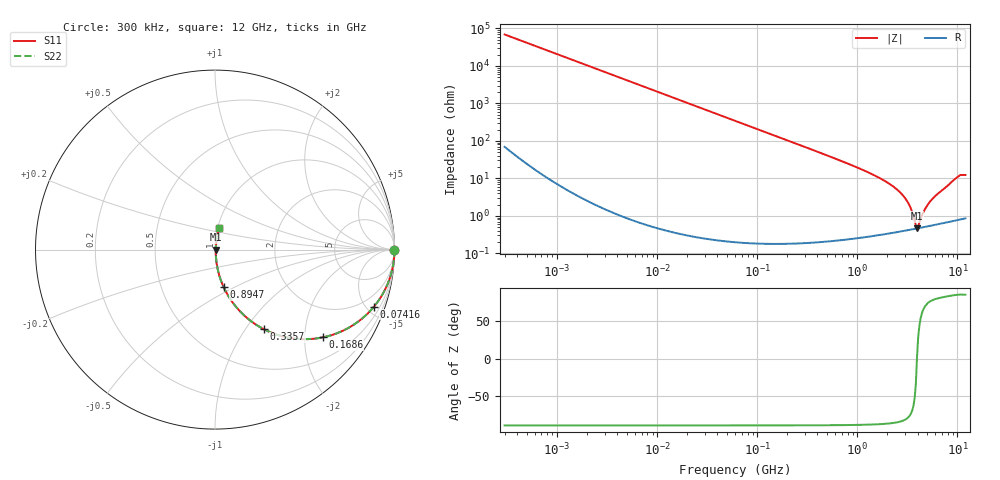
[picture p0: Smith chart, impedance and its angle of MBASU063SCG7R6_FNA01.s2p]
! MBASU063SCG7R6_FNA01  S-PARAMETER MODEL  ( General Type )
! Model Generated by TAIYO YUDEN Corporation (http://www.ty-top.com)
! Version 1.0
! TAIYO YUDEN Control No. 130801
! Copyright(c) 2013 TAIYO YUDEN CO.,LTD. All Rights Reserved.
! Product Description (link to TY-COMPAS)
! https://ds.yuden.co.jp/TYCOMPAS/or/detail?pn=MBASU063SCG7R6DFNA01&u=M
! Products Name : Multilayer Ceramic Capacitors
! Characteristics :
!  Capacitance : 7.6 pF , Rated Voltage : 50V , TCC : CG / C0G
!  Case Size : 0.6 x 0.3 / 0.024 x 0.012 [mm/inch] , Thickness : 0.3 / 0.012 [mm/inch]
!  (Conditions: Temperature = 25 degC , DC Bias Current/Voltage = 0A / 0V)
! External Node Assignments :
!  1  o---| |---o  2
! GND o---------o GND
! Frequency Range : 0.3MHz  -  12000MHz  [ 401 STEP ]
# MHz S RI R 50
! Freq[MHz].  S11 Real  S11 Imag  S21 Real  S21 Imag  S12 Real  S12 Imag  S22 Real  S22 Imag
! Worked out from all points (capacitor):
!   401 points, 300 kHz to 12 GHz, reference 50 ohm
!   read as one part in series: C = 7.68 pF near 316.3 kHz
!   lowest |Z| = 460 mohm at 3.944 GHz (marker M1)
!   series resonance near 3.94 GHz, so ESL is about 210 pH
!   S11 on the Smith chart (normalised r, x): 300 kHz: open; 74.16 MHz: 1.00, -5.59; 168.6 MHz: 1.00, -2.45; 335.7 MHz: 1.00, -1.23; 894.7 MHz: 1.00, -0.44; 12 GHz: 1.02, +0.25
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0.3  1 -0.00145  3.55e-06 0.00145  3.55e-06 0.00145  1 -0.00145
1.769972  0.9999 -0.00854  7.51e-05 0.00854  7.51e-05 0.00854  0.9999 -0.00854
10.44266  0.9975 -0.0503  0.00255 0.0503  0.00255 0.0503  0.9975 -0.0503
27.10171  0.9831 -0.1286  0.0169 0.1286  0.0169 0.1286  0.9831 -0.1286
60  0.9225 -0.2672  0.0775 0.2672  0.0775 0.2672  0.9225 -0.2672
74.16388  0.8862 -0.3173  0.1138 0.3173  0.1138 0.3173  0.8862 -0.3173
168.5979  0.6006 -0.4891  0.3994 0.4891  0.3994 0.4891  0.6006 -0.4891
335.7268  0.2736 -0.4442  0.7264 0.4442  0.7264 0.4442  0.2736 -0.4442
353.9943  0.2528 -0.433  0.7472 0.433  0.7472 0.433  0.2528 -0.433
540.8523  0.1252 -0.3282  0.8748 0.3282  0.8748 0.3282  0.1252 -0.3282
894.6982  0.0481 -0.2086  0.9519 0.2086  0.9519 0.2086  0.0481 -0.2086
2088.533  0.00841 -0.0707  0.9916 0.0707  0.9916 0.0707  0.00841 -0.0707
2581.562  0.00581 -0.0456  0.9942 0.0456  0.9942 0.0456  0.00581 -0.0456
3026.31  0.0048 -0.0281  0.9952 0.0281  0.9952 0.0281  0.0048 -0.0281
3364.605  0.00451 -0.0168  0.9955 0.0168  0.9955 0.0168  0.00451 -0.0168
3740.715  0.00449 -0.00576  0.9955 0.00576  0.9955 0.00576  0.00449 -0.00576
3944.255  0.00458 0.000122  0.9954 -0.000122  0.9954 -0.000122  0.00458 0.000122
4158.869  0.00472 0.00439  0.9953 -0.00439  0.9953 -0.00439  0.00472 0.00439
4875.354  0.00537 0.0161  0.9946 -0.0161  0.9946 -0.0161  0.00537 0.0161
5715.274  0.00639 0.0286  0.9936 -0.0286  0.9936 -0.0286  0.00639 0.0286
9968.853  0.0187 0.1042  0.9813 -0.1042  0.9813 -0.1042  0.0187 0.1042
12000  0.023 0.1189  0.977 -0.1189  0.977 -0.1189  0.023 0.1189
